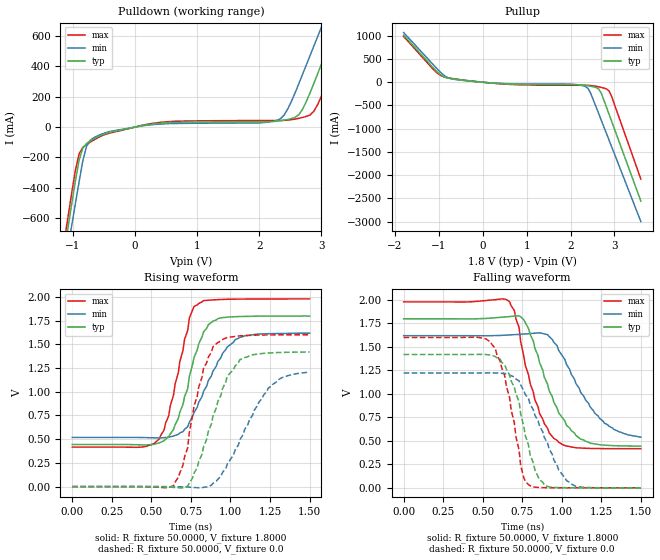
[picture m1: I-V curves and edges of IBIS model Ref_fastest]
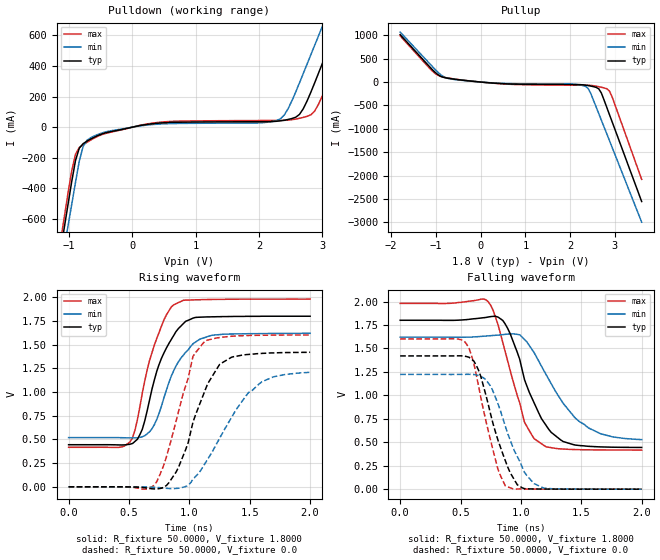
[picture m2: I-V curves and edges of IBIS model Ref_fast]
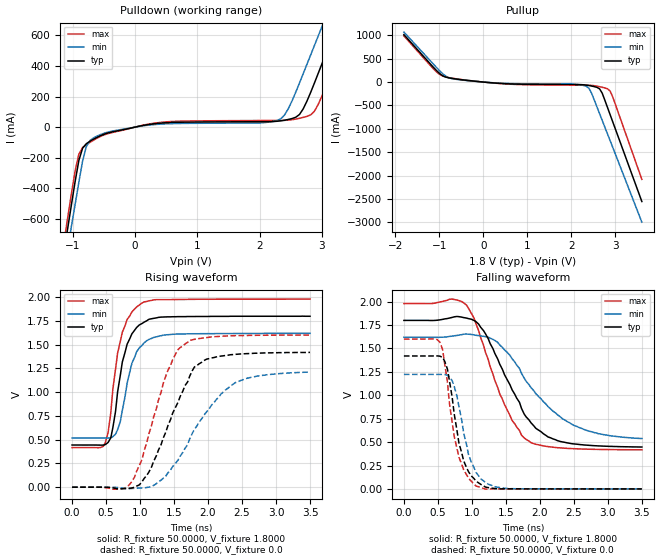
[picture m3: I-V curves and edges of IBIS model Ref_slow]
| Integrated Devices Technolgy, Inc
[IBIS Ver]   4.2
[File name]   9fgv0831.ibs
[File Rev]   1.4
|Rev history   1.4   Update Ref models with different slew-rate setting 08-17-2015
|Rev history   1.3   Update LP_HCSL models with 0v6,0v7,0v8,0v9 08-05-2015
|Rev history   1.2   update LP_HCSL model
|Rev history   1.1   update IN data
|Rev history   1.0   original ibis data
[Date]   17 Aug, 2015
[Disclaimer] Integrated Device Technology, Inc. ("IDT") hereby grants the
   user of this ibis model a non-exclusive, nontransferable
   license to use this ibis model under the following terms. the
   user is granted this license only to use the ibis model and is
   not granted rights to sell, copy (except as needed to run the
   ibis model), rent, lease or sub-license the ibis model in
   whole or in part, or in modified form to anyone. the user may
   modify the ibis model to suit its specific applications, but
   rights to derivative works and such modifications shall belong
   to idt. this ibis model is provided on an as is" basis and idt
   makes absolutely no warranty with respect to the information
   contained herein. idt disclaims and customer waives all
   warranties, express and implied, including warranties of
   merchantability and fitness for a particular purpose. the
   entire risk as to quality and performance is with the user
   accordingly, in no event shall idt be liable for any direct or
   indirect damages, whether in contract or tort, including any
   lost profits or other incidental, consequential, exemplary, or
   punitive damages arising out of the use or application of the
   ibis model. further, idt reserves the right to make changes
   without notice to any product herein to improve reliability,
   function, or design. idt does not convey any license under
   patent rights or any other intellectual property rights,
   including those of third parties. idt is not obligated to
   provide maintenance or support for the licensed ibis model.
[Copyright]   Copyright 2012, Integrated Devices Technolgy, Inc. all rights
   reserved
[Component]   9FGV0831
[Manufacturer] Integrated Device Technology, Inc.
[Package]
R_pkg   72.4655m   58.886m   86.045m
L_pkg   1.47175nH   1.11650nH   1.77850nH
C_pkg   0.07747pF   0.07444pF   0.08050pF
[Pin] signal_name  model_name
1   vSS_EN_tri   GND
2   GNDXTAL   GND
3   X1_25   NC
4   X2   NC
5   VDDXTAL1.8   POWER
6   VDDREF1.8   POWER
7   vSADR/REF1.8   REF
8   GNDREF   GND
9   GNDDIG   GND
10   SCLK_3.3   SCIN
11   SDATA_3.3   SCIN
12   VDDDIG1.8   POWER
13   VDDIO   POWER
14   vOE0#   IN
15   DIF0   LP_HCSL
16   DIF0#   LP_HCSL
17   vOE1#   IN
18   DIF1   LP_HCSL
19   DIF1#   LP_HCSL
20   VDDA1.8   POWER
21   VDDIO   POWER
22   GND   GND
23   DIF2   LP_HCSL
24   DIF2#   LP_HCSL
25   vOE2#   IN
26   DIF3   LP_HCSL
27   DIF3#   LP_HCSL
28   vOE3#   IN
29   GND   GND
30   VDDA1.8   POWER
31   VDDIO   POWER
32   DIF4   LP_HCSL
33   DIF4#   LP_HCSL
34   vOE4#   IN
35   DIF5   LP_HCSL
36   DIF5#   LP_HCSL
37   vOE5#   IN
38   VDDA1.8   POWER
39   VDDIO   POWER
40   GND   GND
41   DIF6   LP_HCSL
42   DIF6#   LP_HCSL
43   vOE6#   IN
44   DIF7   LP_HCSL
45   DIF7#   LP_HCSL
46   vOE7#   IN
47   VDDIO   POWER
48   ^CKPWRGD_PD#   PD
[Diff Pin]  inv_pin  vdiff tdelay_typ tdelay_min  tdelay_max
15   16   NA   0   0   0
18   19   NA   0   0   0
23   24   NA   0   0   0
26   27   NA   0   0   0
32   33   NA   0   0   0
35   36   NA   0   0   0
41   42   NA   0   0   0
44   45   NA   0   0   0
[Model Selector] LP_HCSL
lphcsl_0v6_fast amplitude 0.6V, slew rate fast
lphcsl_0v6_slow amplitude 0.6V, slew rate slow
lphcsl_0v7_fast amplitude 0.7V, slew rate fast
lphcsl_0v7_slow amplitude 0.7V, slew rate slow
lphcsl_0v8_fast amplitude 0.8V, slew rate fast
lphcsl_0v8_slow amplitude 0.8V, slew rate slow
lphcsl_0v9_fast amplitude 0.9V, slew rate fast
lphcsl_0v9_slow amplitude 0.9V, slew rate slow
[Model Selector] REF
Ref_fastest amplitude, slew rate fastest
Ref_fast amplitude, slew rate fast
Ref_slow amplitude, slew rate slow
Ref_slowest amplitude, slew rate slowest
| Models and submodels in the file (15): Ref_fastest (Output), Ref_fast (Output), Ref_slow (Output), Ref_slowest (Output), lphcsl_0v6_fast (Output), lphcsl_0v6_slow (Output), lphcsl_0v7_fast (Output), lphcsl_0v7_slow (Output), lphcsl_0v8_fast (Output), lphcsl_0v8_slow (Output), lphcsl_0v9_fast (Output), lphcsl_0v9_slow (Output), SCIN (Input), IN (Input), PD (Input)
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|   Model Ref_fastest
[Model]  Ref_fastest
Model_type Output
Polarity   Non-Inverting
Enable   Active-High
Vmeas =  0.9000V
Cref =   5.0000pF
Rref =   0.0
Vref =   0.9000V
C_comp   1.1000pF   1.0000pF   1.2000pF
[Temperature Range]   25.0000   75.0000   0.0
[Voltage Range]   1.8000V   1.6200V   1.9800V
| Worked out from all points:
|   slope of the pulldown table from 0 to 0.27 V, typ, clamps not added: 13.6 ohm
|   slope of the pullup table from 0 to 0.27 V, typ, clamps not added: 12.6 ohm
|   rising waveform, R_fixture 50.0000, V_fixture 1.8000: 20-80 % time 136ps typ, 189ps min, 126ps max; typ from 0.444 V to 1.8 V
|   rising waveform, R_fixture 50.0000, V_fixture 0.0: 20-80 % time 171ps typ, 228ps min, 129ps max; typ from 0 V to 1.42 V
|   falling waveform, R_fixture 50.0000, V_fixture 1.8000: 20-80 % time 193ps typ, 229ps min, 148ps max; typ from 1.8 V to 0.445 V
|   falling waveform, R_fixture 50.0000, V_fixture 0.0: 20-80 % time 136ps typ, 191ps min, 115ps max; typ from 1.42 V to 0 V
[Pulldown]
|Voltage   I(typ)   I(min)   I(max)
-1.8V     -2.523A    -2.538A    -2.518A
-1.14V    -819.8mA   -941.4mA   -756.5mA
-1.02V    -510.3mA   -651.3mA   -436.5mA
-900mV    -218.2mA   -361.2mA   -176.9mA
-780mV    -108.3mA   -127.1mA   -115.2mA
-480mV    -44.15mA   -37.97mA   -48.5mA
2.28V     38.45mA    43.47mA    43.55mA
2.82V     227.8mA    473.1mA    80.46mA
3V        414.1mA    657.2mA    202.9mA
3.24V     664.6mA    902.8mA    452mA
3.42V     852.6mA    1.087A     641.9mA
3.6V      1.04A      1.271A     832mA
[Pullup]
|Voltage   I(typ)   I(min)   I(max)
-1.8V     1.013A     1.068A     986.3mA
-1.08V    265.2mA    331.9mA    235.3mA
-900mV    125.7mA    162.8mA    121.5mA
-780mV    89.6mA     91.86mA    94.5mA
600mV     -39.1mA    -31.81mA   -45.18mA
2.04V     -52.88mA   -43.73mA   -64.93mA
2.28V     -59.25mA   -73.36mA   -65.86mA
2.4V      -74.81mA   -134.8mA   -67.72mA
2.64V     -144.9mA   -673.4mA   -99.02mA
2.7V      -237.1mA   -818.3mA   -112.1mA
2.88V     -697mA     -1.253A    -192.5mA
3.6V      -2.555A    -2.996A    -2.081A
[Ramp]
| variable   typ   min   max
dV/dt_r  0.8514/0.1699n   0.7242/0.2234n   0.9606/0.1420n
dV/dt_f  0.8132/0.1864n   0.6479/0.2269n   0.9379/0.1594n
R_load = 50.0000
[Rising Waveform]
R_fixture= 50.0000
V_fixture= 1.8000
V_fixture_min= 1.6200
V_fixture_max= 1.9800
|time   V(typ)   V(min)   V(max)
0s        443.8mV    518.8mV    416.8mV
440ps     440.3mV    517.6mV    416.8mV
550ps     460.4mV    513.6mV    503.1mV
610ps     527mV      519.6mV    749.6mV
670ps     716.4mV    550.3mV    1.2V
740ps     1.163V     677.9mV    1.777V
800ps     1.509V     892.4mV    1.932V
890ps     1.745V     1.219V     1.97V
1.03ns    1.792V     1.549V     1.977V
1.5ns     1.799V     1.618V     1.98V
[Rising Waveform]
R_fixture= 50.0000
V_fixture= 0.0
V_fixture_min= 0.0
V_fixture_max= 0.0
|time   V(typ)   V(min)   V(max)
0s        0V         0V         0V
640ps     -8.307mV   -1.069mV   8.636mV
700ps     -12.45mV   -2.881mV   226.7mV
760ps     89.6mV     -8.52mV    742mV
830ps     419.3mV    -8.047mV   1.25V
880ps     663.7mV    14.63mV    1.42V
980ps     1.165V     237.2mV    1.574V
1.06ns    1.34V      494.6mV    1.59V
1.24ns    1.409V     1.04V      1.6V
1.5ns     1.419V     1.207V     1.601V
[Falling Waveform]
R_fixture= 50.0000
V_fixture= 1.8000
V_fixture_min= 1.6200
V_fixture_max= 1.9800
|time   V(typ)   V(min)   V(max)
0s        1.8V       1.62V      1.98V
650ps     1.821V     1.626V     2.004V
700ps     1.828V     1.631V     1.89V
760ps     1.789V     1.638V     1.402V
860ps     1.33V      1.65V      789.1mV
950ps     911.1mV    1.549V     526.1mV
1.09ns    557.9mV    1.109V     426.2mV
1.21ns    466.6mV    791.9mV    418.9mV
1.33ns    448.5mV    621.7mV    417.4mV
1.5ns     444.6mV    540.2mV    416.9mV
[Falling Waveform]
R_fixture= 50.0000
V_fixture= 0.0
V_fixture_min= 0.0
V_fixture_max= 0.0
|time   V(typ)   V(min)   V(max)
0s        1.42V      1.223V     1.601V
550ps     1.414V     1.224V     1.551V
610ps     1.371V     1.222V     1.348V
670ps     1.2V       1.202V     963.2mV
730ps     918mV      1.138V     402.1mV
740ps     789mV      1.097V     239mV
800ps     351.2mV    890.4mV    22.4mV
890ps     32.24mV    536mV      2.013mV
1.03ns    1.422mV    76.71mV    417uV
1.5ns     -30.7uV    135.3uV    -41.41uV
|   Model Ref_fast
[Model]  Ref_fast
Model_type Output
Polarity   Non-Inverting
Enable   Active-High
Vmeas =  0.9000V
Cref =   5.0000pF
Rref =   0.0
Vref =   0.9000V
C_comp   1.1000pF   1.0000pF   1.2000pF
[Temperature Range]   25.0000   75.0000   0.0
[Voltage Range]   1.8000V   1.6200V   1.9800V
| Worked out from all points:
|   slope of the pulldown table from 0 to 0.27 V, typ, clamps not added: 13.6 ohm
|   slope of the pullup table from 0 to 0.27 V, typ, clamps not added: 12.6 ohm
|   rising waveform, R_fixture 50.0000, V_fixture 1.8000: 20-80 % time 204ps typ, 219ps min, 188ps max; typ from 0.444 V to 1.8 V
|   rising waveform, R_fixture 50.0000, V_fixture 0.0: 20-80 % time 240ps typ, 346ps min, 202ps max; typ from 0 V to 1.42 V
|   falling waveform, R_fixture 50.0000, V_fixture 1.8000: 20-80 % time 241ps typ, 328ps min, 198ps max; typ from 1.8 V to 0.445 V
|   falling waveform, R_fixture 50.0000, V_fixture 0.0: 20-80 % time 195ps typ, 218ps min, 168ps max; typ from 1.42 V to 0 V
[Pulldown]
|Voltage   I(typ)   I(min)   I(max)
-1.8V     -2.523A    -2.538A    -2.518A
-1.14V    -819.8mA   -941.4mA   -756.5mA
-1.02V    -510.3mA   -651.3mA   -436.5mA
-900mV    -218.2mA   -361.2mA   -176.9mA
-780mV    -108.3mA   -127.1mA   -115.2mA
-480mV    -44.15mA   -37.97mA   -48.5mA
2.28V     38.45mA    43.47mA    43.55mA
2.82V     227.8mA    473.1mA    80.46mA
3V        414.1mA    657.2mA    202.9mA
3.24V     664.6mA    902.8mA    452mA
3.42V     852.6mA    1.087A     641.9mA
3.6V      1.04A      1.271A     832mA
[Pullup]
|Voltage   I(typ)   I(min)   I(max)
-1.8V     1.013A     1.068A     986.3mA
-1.08V    265.2mA    331.9mA    235.3mA
-900mV    125.7mA    162.8mA    121.5mA
-780mV    89.6mA     91.86mA    94.5mA
600mV     -39.1mA    -31.81mA   -45.18mA
2.04V     -52.88mA   -43.73mA   -64.93mA
2.28V     -59.25mA   -73.36mA   -65.86mA
2.4V      -74.81mA   -134.8mA   -67.72mA
2.64V     -144.9mA   -673.4mA   -99.02mA
2.7V      -237.1mA   -818.3mA   -112.1mA
2.88V     -697mA     -1.253A    -192.5mA
3.6V      -2.555A    -2.996A    -2.081A
[Ramp]
| variable   typ   min   max
dV/dt_r  0.8514/0.2601n   0.7248/0.3457n   0.9606/0.2140n
dV/dt_f  0.8132/0.2605n   0.6551/0.3282n   0.9378/0.2162n
R_load = 50.0000
[Rising Waveform]
R_fixture= 50.0000
V_fixture= 1.8000
V_fixture_min= 1.6200
V_fixture_max= 1.9800
|time   V(typ)   V(min)   V(max)
0s        443.8mV    518.8mV    416.8mV
510ps     449.7mV    515.9mV    474.9mV
550ps     479.4mV    515.6mV    598.1mV
610ps     605.5mV    527.7mV    986.2mV
690ps     1.028V     612.2mV    1.413V
770ps     1.358V     855.5mV    1.697V
870ps     1.595V     1.224V     1.919V
1.03ns    1.779V     1.508V     1.971V
1.19ns    1.793V     1.599V     1.976V
2ns       1.799V     1.619V     1.98V
[Rising Waveform]
R_fixture= 50.0000
V_fixture= 0.0
V_fixture_min= 0.0
V_fixture_max= 0.0
|time   V(typ)   V(min)   V(max)
0s        0V         0V         0V
710ps     -22.17mV   -4.968mV   18.74mV
790ps     -1.975mV   -13.86mV   234.7mV
890ps     155.1mV    -17.27mV   693mV
1.03ns    682.3mV    78.89mV    1.377V
1.13ns    1.017V     246.4mV    1.54V
1.25ns    1.29V      510.3mV    1.574V
1.49ns    1.396V     993.4mV    1.596V
1.7ns     1.412V     1.161V     1.6V
2ns       1.419V     1.208V     1.601V
[Falling Waveform]
R_fixture= 50.0000
V_fixture= 1.8000
V_fixture_min= 1.6200
V_fixture_max= 1.9800
|time   V(typ)   V(min)   V(max)
0s        1.8V       1.62V      1.98V
710ps     1.83V      1.632V     2.019V
770ps     1.842V     1.638V     1.906V
870ps     1.76V      1.65V      1.465V
990ps     1.384V     1.645V     921.1mV
1.03ns    1.166V     1.593V     712mV
1.11ns    917.8mV    1.454V     537.8mV
1.25ns    606.2mV    1.126V     442.6mV
1.49ns    464.5mV    715.2mV    420.6mV
2ns       444.6mV    528.2mV    417mV
[Falling Waveform]
R_fixture= 50.0000
V_fixture= 0.0
V_fixture_min= 0.0
V_fixture_max= 0.0
|time   V(typ)   V(min)   V(max)
0s        1.42V      1.223V     1.601V
550ps     1.413V     1.224V     1.546V
630ps     1.32V      1.217V     1.22V
710ps     1.002V     1.165V     727.9mV
810ps     522.3mV    910.5mV    210.9mV
870ps     306.6mV    674.7mV    36.78mV
970ps     46.51mV    347.8mV    1.851mV
1.03ns    5.47mV     177.8mV    1.494mV
1.19ns    1.173mV    10.74mV    452.2uV
2ns       10.04uV    50.45uV    1.537uV
|   Model Ref_slow
[Model]  Ref_slow
Model_type Output
Polarity   Non-Inverting
Enable   Active-High
Vmeas =  0.9000V
Cref =   5.0000pF
Rref =   0.0
Vref =   0.9000V
C_comp   1.1000pF   1.0000pF   1.2000pF
[Temperature Range]   25.0000   75.0000   0.0
[Voltage Range]   1.8000V   1.6200V   1.9800V
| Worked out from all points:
|   slope of the pulldown table from 0 to 0.27 V, typ, clamps not added: 13.6 ohm
|   slope of the pullup table from 0 to 0.27 V, typ, clamps not added: 12.6 ohm
|   rising waveform, R_fixture 50.0000, V_fixture 1.8000: 20-80 % time 205ps typ, 215ps min, 201ps max; typ from 0.444 V to 1.8 V
|   rising waveform, R_fixture 50.0000, V_fixture 0.0: 20-80 % time 506ps typ, 669ps min, 408ps max; typ from 0 V to 1.42 V
|   falling waveform, R_fixture 50.0000, V_fixture 1.8000: 20-80 % time 572ps typ, 744ps min, 484ps max; typ from 1.8 V to 0.448 V
|   falling waveform, R_fixture 50.0000, V_fixture 0.0: 20-80 % time 214ps typ, 236ps min, 208ps max; typ from 1.42 V to 0 V
[Pulldown]
|Voltage   I(typ)   I(min)   I(max)
-1.8V     -2.523A    -2.538A    -2.518A
-1.14V    -819.8mA   -941.4mA   -756.5mA
-1.02V    -510.3mA   -651.3mA   -436.5mA
-900mV    -218.2mA   -361.2mA   -176.9mA
-780mV    -108.3mA   -127.1mA   -115.2mA
-480mV    -44.15mA   -37.97mA   -48.5mA
2.28V     38.45mA    43.47mA    43.55mA
2.82V     227.8mA    473.1mA    80.46mA
3V        414.1mA    657.2mA    202.9mA
3.24V     664.6mA    902.8mA    452mA
3.42V     852.6mA    1.087A     641.9mA
3.6V      1.04A      1.271A     832mA
[Pullup]
|Voltage   I(typ)   I(min)   I(max)
-1.8V     1.013A     1.068A     986.3mA
-1.08V    265.2mA    331.9mA    235.3mA
-900mV    125.7mA    162.8mA    121.5mA
-780mV    89.6mA     91.86mA    94.5mA
600mV     -39.1mA    -31.81mA   -45.18mA
2.04V     -52.88mA   -43.73mA   -64.93mA
2.28V     -59.25mA   -73.36mA   -65.86mA
2.4V      -74.81mA   -134.8mA   -67.72mA
2.64V     -144.9mA   -673.4mA   -99.02mA
2.7V      -237.1mA   -818.3mA   -112.1mA
2.88V     -697mA     -1.253A    -192.5mA
3.6V      -2.555A    -2.996A    -2.081A
[Ramp]
| variable   typ   min   max
dV/dt_r  0.8514/0.5070n   0.7272/0.6958n   0.9606/0.4068n
dV/dt_f  0.8114/0.6020n   0.6491/0.7746n   0.9372/0.4823n
R_load = 50.0000
[Rising Waveform]
R_fixture= 50.0000
V_fixture= 1.8000
V_fixture_min= 1.6200
V_fixture_max= 1.9800
|time   V(typ)   V(min)   V(max)
0s        443.8mV    518.8mV    416.8mV
490ps     449.1mV    517.3mV    471.1mV
570ps     520.1mV    519.4mV    782.9mV
600ps     625.8mV    531.9mV    1.031V
670ps     1.003V     606.2mV    1.411V
740ps     1.319V     811.1mV    1.632V
880ps     1.614V     1.304V     1.844V
1.03ns    1.723V     1.493V     1.939V
1.48ns    1.794V     1.609V     1.975V
3.5ns     1.799V     1.619V     1.98V
[Rising Waveform]
R_fixture= 50.0000
V_fixture= 0.0
V_fixture_min= 0.0
V_fixture_max= 0.0
|time   V(typ)   V(min)   V(max)
0s        0V         0V         0V
850ps     -11.15mV   -15.32mV   31.71mV
1.03ns    58.14mV    -8.151mV   293.1mV
1.13ns    159.3mV    1.123mV    561mV
1.41ns    647.8mV    151mV      1.229V
1.56ns    896mV      286.1mV    1.45V
1.73ns    1.168V     508.4mV    1.544V
1.98ns    1.348V     793.7mV    1.575V
2.4ns     1.398V     1.1V       1.595V
3.5ns     1.419V     1.212V     1.601V
[Falling Waveform]
R_fixture= 50.0000
V_fixture= 1.8000
V_fixture_min= 1.6200
V_fixture_max= 1.9800
|time   V(typ)   V(min)   V(max)
0s        1.8V       1.62V      1.98V
710ps     1.832V     1.632V     2.028V
920ps     1.825V     1.654V     1.965V
1.17ns    1.692V     1.63V      1.538V
1.48ns    1.22V      1.485V     900.2mV
1.73ns    860mV      1.235V     574.3mV
1.87ns    705.9mV    1.082V     494.5mV
2.12ns    555.3mV    879.6mV    452.1mV
2.51ns    480.3mV    676mV      429.5mV
3.5ns     447.7mV    538.1mV    418mV
[Falling Waveform]
R_fixture= 50.0000
V_fixture= 0.0
V_fixture_min= 0.0
V_fixture_max= 0.0
|time   V(typ)   V(min)   V(max)
0s        1.42V      1.223V     1.601V
530ps     1.418V     1.223V     1.567V
570ps     1.404V     1.223V     1.488V
640ps     1.281V     1.215V     1.145V
740ps     801.7mV    1.097V     561.4mV
810ps     488.3mV    878.8mV    337.1mV
950ps     184.9mV    369.3mV    114.6mV
1.06ns    83.76mV    177.1mV    31.61mV
1.52ns    1.661mV    4.843mV    759.4uV
3.5ns     21.09uV    39.51uV    -24.76uV
